FUNCTION_BLOCK FB_TxtParser					(* stAcquisitionData Data Parser *)
VAR_INPUT
	bExecute	: BOOL;
	sFilePathSource			: T_MaxString;
	sFilePathDestination	: T_MaxString;
	eMode		: INT;		(* chose Datatype *)

	nParsePerCycle	: INT := nAcquisitionBlock;	(* in this case , must = nAcquisitionBlock*)
END_VAR
VAR_OUTPUT
 	bBusy	:	BOOL;
	bError	:	BOOL;
	nErrId	:	UDINT;

END_VAR
VAR
	iSeq : INT;	
	iExceptionSeq	: INT;	
	(* 0:Source  ; 1:Destination  *)
	fbFileOpen		: ARRAY [0..1] OF FB_FileOpen;
	fbFileSeek		: ARRAY [0..1] OF  FB_FileSeek;
	fbFileRead		: ARRAY [0..1] OF  FB_FileRead;
	fbFileWrite		: ARRAY [0..1] OF  FB_FileWrite;
	fbFileClose		: ARRAY [0..1] OF  FB_FileClose;

	GetBuffer		: ARRAY [0..65535] OF BYTE;		(* Source bin data *)	
	PutBuffer		: ARRAY [0..65535] OF BYTE;		(* Text info data buffer *)

	i 				: INT;
	pPutPointer		: POINTER TO T_MaxString;
	pMountAcuData	: POINTER TO stAcquisitionData;

	nGetSeeker		: UDINT;	
	nPutSeeker		: UDINT;
END_VAR


CASE iSeq OF
0:
	IF bExecute THEN
		bBusy := TRUE;
		iSeq := iSeq + 1;
	END_IF
	//iSeq := 0;
1:	(* Open source file *)
	fbFileOpen[0](sNetId:= sFileTargetNetId,			(* Access target id  *)
		sPathName:= sFilePathSource,	(* Access Path *)
		nMode:= FOPEN_MODEBINARY OR FOPEN_MODEREAD,		(* Binary Format & Read Mode  *)
		ePath:= PATH_GENERIC,
		bExecute:= TRUE,
		tTimeout:= DEFAULT_ADS_TIMEOUT,
		bBusy=> ,
		bError=> ,
		nErrId=> ,
		hFile=> );
		
	IF 	NOT(fbFileOpen[0].bBusy) AND NOT(fbFileOpen[0].bError) THEN
		fbFileOpen[0](bExecute:= FALSE);
		iSeq := iSeq + 1;
	ELSIF fbFileOpen[0].bError THEN
		fbFileOpen[0](bExecute:= FALSE);
		iExceptionSeq := iSeq;
		iSeq := 999;
	END_IF
2:	(* Open Destination file *)
	fbFileOpen[1](sNetId:= sFileTargetNetId,			(* Access target id  *)
		sPathName:= sFilePathDestination,	(* Access Path *)
		nMode:= FOPEN_MODEBINARY OR FOPEN_MODEWRITE,		(* Binary Format & Write Mode & Overrite contents   *)
		ePath:= PATH_GENERIC,
		bExecute:= TRUE,
		tTimeout:= DEFAULT_ADS_TIMEOUT,
		bBusy=> ,
		bError=> ,
		nErrId=> ,
		hFile=> );
		
	IF 	NOT(fbFileOpen[01].bBusy) AND NOT(fbFileOpen[1].bError) THEN
		fbFileOpen[1](bExecute:= FALSE);
		iSeq := iSeq + 1;
	ELSIF fbFileOpen[1].bError THEN
		fbFileOpen[1](bExecute:= FALSE);
		iExceptionSeq := iSeq;
		iSeq := 999;
	END_IF
3:	(* Seek to Start position *)
	nGetSeeker := SIZEOF(PRG_DatFileCreat.DatHeader);		(* Give File seeker position *)
	nPutSeeker := 0;					(* Put seeker from 0 *)	
	fbFileSeek[0](sNetId:= sFileTargetNetId, 
		hFile:= fbFileOpen[0].hFile, 
		nSeekPos:= nGetSeeker, 		(* Seek to record start position *)
		eOrigin:= SEEK_SET, 
		bExecute:= TRUE, 
		tTimeout:= DEFAULT_ADS_TIMEOUT, 
		bBusy=> , 
		bError=> , 
		nErrId=> );
		
	IF NOT(fbFileSeek[0].bBusy) AND NOT(fbFileSeek[0].bError) THEN
		fbFileSeek[0](bExecute:= FALSE);
		iSeq := 10;
	ELSIF fbFileSeek[0].bError THEN
		fbFileSeek[0](bExecute:= FALSE);
		iExceptionSeq := iSeq;
		iSeq := 999;
	END_IF
10:		(* Get Data *)
	fbFileRead[0](sNetId:= sFileTargetNetId, 
		hFile:= fbFileOpen[0].hFile, 
		pReadBuff:= ADR(GetBuffer), 
		cbReadLen:= SIZEOF(PRG_DatFileCreat.DatAcqBlock), 		(* Get size = define sizeof(nAcquisitionBlock)  *)
		bExecute:= TRUE, 
		tTimeout:= DEFAULT_ADS_TIMEOUT, 
		bBusy=> , 
		bError=> , 
		nErrId=> , 
		cbRead=> , 
		bEOF=> );

	IF NOT(fbFileRead[0].bBusy) AND NOT(fbFileRead[0].bError) THEN
		IF fbFileRead[0].cbRead <> fbFileRead[0].cbReadLen THEN		(* Check for act read len mach or not *)
			fbFileRead[0](bExecute:= FALSE);
			iExceptionSeq := iSeq;		
			iSeq := 888;			
		ELSE
			fbFileRead[0](bExecute:= FALSE);
			iSeq := iSeq + 1;				
		END_IF

		IF fbFileRead[0].bEOF THEN 	(* meet EoF of source file *)
			fbFileRead[0](bExecute:= FALSE);
			iSeq := 50;				(* goto close sequence *)
		END_IF		
	ELSIF fbFileRead[0].bError THEN
		fbFileRead[0](bExecute:= FALSE);
		iExceptionSeq := iSeq;
		iSeq := 999;
	END_IF
11:	(* Decode Data into PutBuffer *)
	(* Decord layout = stAcquisitionData *)
	pPutPointer := ADR(PutBuffer);		(* Reset pointer to begin *)
	FOR i := 0 TO nAcquisitionBlock BY 1 DO
		pMountAcuData := ADR(GetBuffer) + (i * SIZEOF(pMountAcuData^));

	
		pPutPointer^ := DCTIME_TO_STRING(pMountAcuData^.nDcTimeStamp);		(* First Info , DC TimeStamp *)
		pPutPointer^ := CONCAT(pPutPointer^ , ',');
		pPutPointer := pPutPointer + Len(pPutPointer^);						(* Shift pointer to next Info *)
		
		pPutPointer^ := DINT_TO_STRING(pMountAcuData^.AIN0);			(* Further Acq Data *)
		pPutPointer^ := CONCAT(pPutPointer^ , ',');
		pPutPointer := pPutPointer + Len(pPutPointer^);						(* Shift pointer to next Info *)
	
		pPutPointer^ := DINT_TO_STRING(pMountAcuData^.AIN1);			(* Further Acq Data *)
		pPutPointer^ := CONCAT(pPutPointer^ , ',');
		pPutPointer := pPutPointer + Len(pPutPointer^);						(* Shift pointer to next Info *)
		
		pPutPointer^ := DINT_TO_STRING(pMountAcuData^.AIN2);			(* Further Acq Data *)
		pPutPointer^ := CONCAT(pPutPointer^ , ',');
		pPutPointer := pPutPointer + Len(pPutPointer^);						(* Shift pointer to next Info *)

		pPutPointer^ := DINT_TO_STRING(pMountAcuData^.AIN3);			(* Further Acq Data *)
		pPutPointer^ := CONCAT(pPutPointer^ , ',');
		pPutPointer := pPutPointer + Len(pPutPointer^);						(* Shift pointer to next Info *)

		pPutPointer^ := UINT_TO_STRING(pMountAcuData^.ADC_nSample);			(* Further Acq Data *)
		pPutPointer^ := CONCAT(pPutPointer^ , ',');
		pPutPointer := pPutPointer + Len(pPutPointer^);						(* Shift pointer to next Info *)

		pPutPointer^ := UINT_TO_STRING(pMountAcuData^.ECAT_IRQ_Counter);			(* Further Acq Data *)
		pPutPointer^ := CONCAT(pPutPointer^ , ',');
		pPutPointer := pPutPointer + Len(pPutPointer^);						(* Shift pointer to next Info *)

		pPutPointer^ := UINT_TO_STRING(pMountAcuData^.ECAT_SYNC0_Counter);			(* Further Acq Data *)
		pPutPointer^ := CONCAT(pPutPointer^ , ',');
		pPutPointer := pPutPointer + Len(pPutPointer^);						(* Shift pointer to next Info *)

		pPutPointer^ := UINT_TO_STRING(pMountAcuData^.ECAT_SYNC1_Counter);			(* Further Acq Data *)
		pPutPointer^ := CONCAT(pPutPointer^ , '$0D');		
		pPutPointer^ := CONCAT(pPutPointer^ , '$0A');
		pPutPointer := pPutPointer + Len(pPutPointer^);						(* Shift pointer to next Info *)
	END_FOR
	
	
	nGetSeeker := nGetSeeker + SIZEOF(PRG_DatFileCreat.DatAcqBlock);
	//nPutSeeker := nPutSeeker + (pPutPointer - ADR(PutBuffer));
	iSeq := iSeq + 1;
12:
	fbFileWrite[1](sNetId:= sFileTargetNetId, 
		hFile:= fbFileOpen[1].hFile, 
		pWriteBuff:= ADR(PutBuffer), 
		cbWriteLen:= pPutPointer - ADR(PutBuffer), 
		bExecute:= TRUE, 
		tTimeout:= DEFAULT_ADS_TIMEOUT, 
		bBusy=> , 
		bError=> , 
		nErrId=> , 
		cbWrite=> );
	
	IF NOT(fbFileWrite[1].bBusy) AND NOT(fbFileWrite[1].bError) THEN
		fbFileWrite[1](bExecute:= FALSE);

		nPutSeeker := nPutSeeker + (pPutPointer - ADR(PutBuffer));
		iSeq := iSeq + 1;
	ELSIF fbFileWrite[1].bError THEN
		fbFileWrite[1](bExecute:= FALSE);
		iExceptionSeq := iSeq;
		iSeq := 999;
	END_IF
13:	(* Seek both file *)
	fbFileSeek[0](sNetId:= sFileTargetNetId, 
		hFile:= fbFileOpen[0].hFile, 
		nSeekPos:= nGetSeeker, 		(* Seek to record start position *)
		eOrigin:= SEEK_SET, 
		bExecute:= TRUE, 
		tTimeout:= DEFAULT_ADS_TIMEOUT, 
		bBusy=> , 
		bError=> , 
		nErrId=> );

	fbFileSeek[1](sNetId:= sFileTargetNetId, 
		hFile:= fbFileOpen[1].hFile, 
		nSeekPos:= nPutSeeker, 		(* Seek to record start position *)
		eOrigin:= SEEK_SET, 
		bExecute:= TRUE, 
		tTimeout:= DEFAULT_ADS_TIMEOUT, 
		bBusy=> , 
		bError=> , 
		nErrId=> );
		
	IF (NOT(fbFileSeek[0].bBusy) AND NOT(fbFileSeek[0].bError)) AND (NOT(fbFileSeek[1].bBusy) AND NOT(fbFileSeek[1].bError)) THEN
		fbFileSeek[0](bExecute:= FALSE);
		fbFileSeek[1](bExecute:= FALSE);
		iSeq := 10;
	ELSIF fbFileSeek[0].bError OR fbFileSeek[1].bError  THEN
		fbFileSeek[0](bExecute:= FALSE);
		fbFileSeek[1](bExecute:= FALSE);
		iExceptionSeq := iSeq;
		iSeq := 999;
	END_IF	
50:
	fbFileClose[0](sNetId:= sFileTargetNetId, 
		hFile:= fbFileOpen[0].hFile,  
		bExecute:= TRUE, 
		tTimeout:= DEFAULT_ADS_TIMEOUT, 
		bBusy=> , 
		bError=> , 
		nErrId=> );

	fbFileClose[1](sNetId:= sFileTargetNetId, 
		hFile:= fbFileOpen[1].hFile,  
		bExecute:= TRUE, 
		tTimeout:= DEFAULT_ADS_TIMEOUT, 
		bBusy=> , 
		bError=> , 
		nErrId=> );
	
	IF (NOT(fbFileClose[0].bBusy) AND NOT(fbFileClose[0].bError)) AND (NOT(fbFileClose[1].bBusy) AND NOT(fbFileClose[1].bError)) THEN
		fbFileClose[0](bExecute:= FALSE);
		fbFileClose[1](bExecute:= FALSE);
		bBusy := FALSE;
		iSeq := iSeq + 1;
	ELSIF fbFileSeek[1].bError THEN
		fbFileClose[0](bExecute:= FALSE);
		fbFileClose[1](bExecute:= FALSE);
		iExceptionSeq := iSeq;
		iSeq := 999;
	END_IF
51:
	IF NOT(bExecute) THEN
		iSeq := 0;
	END_IF

END_CASE


(*

	fbFileOpen[0](sNetId:= sFileTargetNetId,			(* Access target id  *)
		sPathName:= sFilePathSource,	(* Access Path *)
		nMode:= FOPEN_MODEBINARY OR FOPEN_MODEREAD,		(* Binary Format & Read Mode  *)
		ePath:= PATH_GENERIC,
		bExecute:= ,
		tTimeout:= DEFAULT_ADS_TIMEOUT,
		bBusy=> ,
		bError=> ,
		nErrId=> ,
		hFile=> );


	fbFileOpen[1](sNetId:= sFileTargetNetId,			(* Access target id  *)
		sPathName:= sFilePathDestination,	(* Access Path *)
		nMode:= FOPEN_MODEBINARY OR FOPEN_MODEWRITE,		(* Binary Format & Write Mode & Overrite contents   *)
		ePath:= PATH_GENERIC,
		bExecute:= ,
		tTimeout:= DEFAULT_ADS_TIMEOUT,
		bBusy=> ,
		bError=> ,
		nErrId=> ,
		hFile=> );
		
		
		

	fbFileWrite[1](sNetId:= sFileTargetNetId, 
		hFile:= fbFileOpen[1].hFile, 
		pWriteBuff:= ADR(PutBuffer), 
		cbWriteLen:= , 
		bExecute:= , 
		tTimeout:= DEFAULT_ADS_TIMEOUT, 
		bBusy=> , 
		bError=> , 
		nErrId=> , 
		cbWrite=> );


	fbFileSeek[0](sNetId:= sFileTargetNetId, 
		hFile:= fbFileOpen[0].hFile, 
		nSeekPos:= , 		(* Seek to record start position *)
		eOrigin:= SEEK_SET, 
		bExecute:= , 
		tTimeout:= DEFAULT_ADS_TIMEOUT, 
		bBusy=> , 
		bError=> , 
		nErrId=> );

	fbFileSeek[1](sNetId:= sFileTargetNetId, 
		hFile:= fbFileOpen[1].hFile, 
		nSeekPos:= , 		(* Seek to record start position *)
		eOrigin:= SEEK_SET, 
		bExecute:= , 
		tTimeout:= DEFAULT_ADS_TIMEOUT, 
		bBusy=> , 
		bError=> , 
		nErrId=> );

	fbFileRead[0](sNetId:= sFileTargetNetId, 
		hFile:= fbFileOpen[0].hFile, 
		pReadBuff:= ADR(GetBuffer), 
		cbReadLen:= , 		(* Get size = define sizeof(nAcquisitionBlock)  *)
		bExecute:= , 
		tTimeout:= DEFAULT_ADS_TIMEOUT, 
		bBusy=> , 
		bError=> , 
		nErrId=> , 
		cbRead=> , 
		bEOF=> );




	fbFileClose[0](sNetId:= sFileTargetNetId, 
		hFile:= fbFileOpen[0].hFile,  
		bExecute:= , 
		tTimeout:= DEFAULT_ADS_TIMEOUT, 
		bBusy=> , 
		bError=> , 
		nErrId=> );

	fbFileClose[1](sNetId:= sFileTargetNetId, 
		hFile:= fbFileOpen[1].hFile,  
		bExecute:= , 
		tTimeout:= DEFAULT_ADS_TIMEOUT, 
		bBusy=> , 
		bError=> , 
		nErrId=> );
*)

END_FUNCTION_BLOCK
